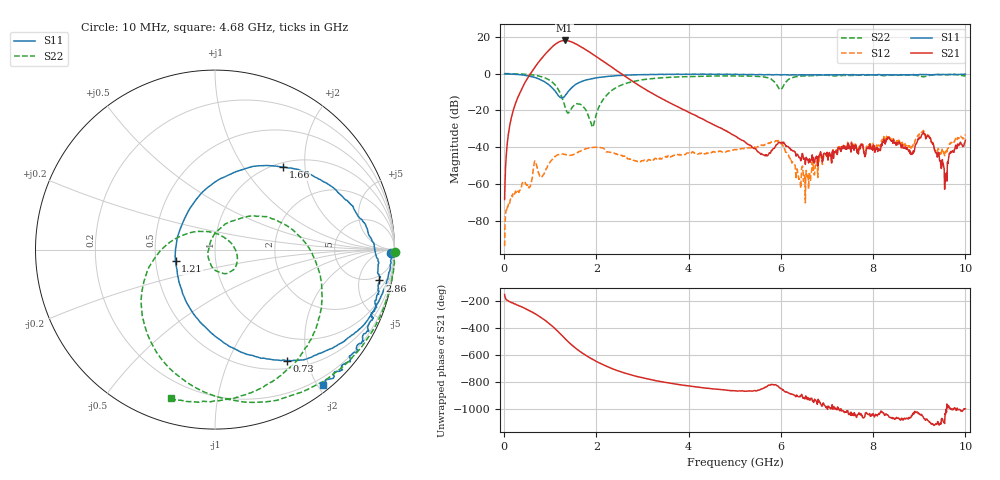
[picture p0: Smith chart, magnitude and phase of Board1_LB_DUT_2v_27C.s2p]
! Created Tue May 27 15:27:29 2025
# hz S ma R 50
! 2 Port Network Data from SP1.SP block
! freq  magS11  angS11  magS21  angS21  magS12  angS12  magS22  angS22
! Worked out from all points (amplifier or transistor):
!   1000 points, 10 MHz to 10 GHz, reference 50 ohm
!   highest |S21| = 18.0 dB at 1.31 GHz (marker M1)
!   |S21| within 3 dB of that: 1.063 GHz to 1.636 GHz (573.1 MHz wide, 42.5 % of centre)
!   unconditionally stable (mu >= 1): 58.5 MHz to 62.27 MHz; 88.9 MHz to 108.3 MHz; 112.2 MHz to end of sweep
!   at 1.67 GHz: K = 7.33, MAG = 16.6 dB, |S12| = -41.9 dB
!   at 5.01 GHz: K = 43.16, MAG = -15.7 dB, |S12| = -41.2 dB
!   at 10 GHz: K = 15.36, MAG = -16.4 dB, |S12| = -33.1 dB
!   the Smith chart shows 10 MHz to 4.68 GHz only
!   S11 on the Smith chart (normalised r, x): 10 MHz: 59, -53; 730 MHz: 0.62, -1.66; 1.21 GHz: 0.64, -0.09; 1.66 GHz: 1.08, +1.55; 2.86 GHz: 4, -9; 4.68 GHz: 0.09, -2.08
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1e7  0.9816 -1.0  0.0003792 -149.5  2.037e-05 177.9  1.005 -0.8
2e8  0.9653 -13.7  0.1028 145.7  0.000566 74.1  0.9959 -17.9
7.3e8  0.7364 -57.2  1.931 55.1  0.002279 58.2  0.878 -75.9
9e8  0.5758 -77.3  3.493 15.2  0.002406 110.0  0.7543 -102.3
1.04e9  0.4126 -101.6  5.328 -23.6  0.004591 100.8  0.591 -130.4
1.13e9  0.305 -126.2  6.591 -52.2  0.005869 87.3  0.4493 -153.3
1.21e9  0.229 -163.8  7.495 -79.5  0.006446 74.3  0.3053 -178.8
1.31e9  0.2395 136.0  7.986 -114.5  0.006377 61.6  0.1389 133.2
1.46e9  0.4068 82.7  7.301 -163.5  0.006106 57.8  0.1148 -1.1
1.66e9  0.5978 50.3  5.421 142.6  0.007949 53.1  0.1449 -67.5
1.68e9  0.6119 48.0  5.237 137.8  0.008126 51.7  0.1389 -71.5
1.88e9  0.724 30.7  3.652 94.8  0.009644 33.2  0.04677 -150.1
2.08e9  0.7964 18.5  2.488 58.1  0.009791 10.8  0.1463 69.8
2.42e9  0.8752 3.2  1.256 8.0  0.006509 -8.2  0.4109 20.1
2.86e9  0.9317 -10.6  0.5386 -38.6  0.004156 -4.0  0.6362 -20.4
3.34e9  0.952 -23.4  0.2361 -74.5  0.004755 10.1  0.7584 -51.0
4.68e9  0.9674 -51.3  0.03388 -137.5  0.00794 -5.8  0.8649 -106.6
5.01e9  0.9683 -57.8  0.02012 -146.7  0.008694 -9.2  0.8679 -118.0
6.67e9  0.931 -90.0  0.005104 158.4  0.002505 162.6  0.8775 -149.0
8.34e9  0.9262 -136.3  0.01863 20.3  0.02034 29.3  0.9023 172.3
9.57e9  0.9491 -168.9  0.001243 37.8  0.006988 55.5  0.9231 162.3
1e10  0.9743 177.4  0.01549 79.6  0.02221 70.2  0.8963 155.9
